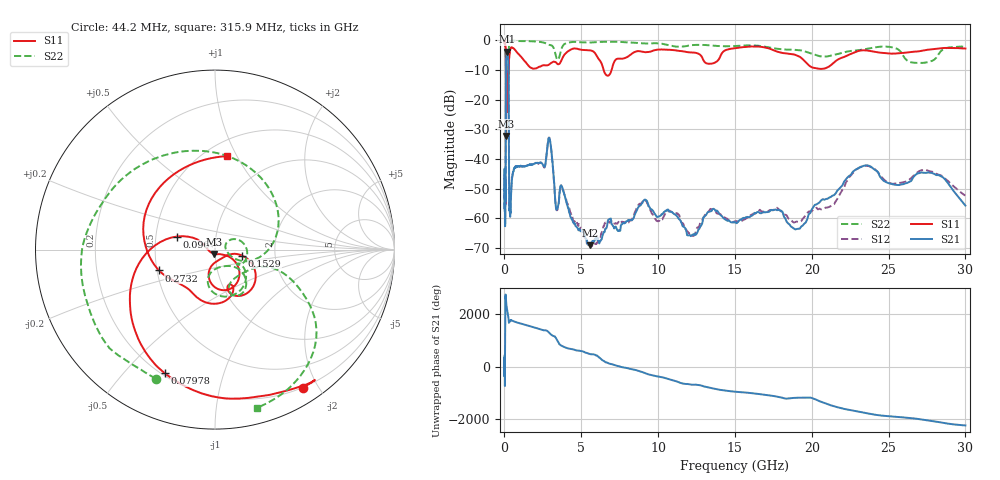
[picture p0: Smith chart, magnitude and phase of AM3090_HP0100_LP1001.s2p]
! Date/Time: Thu, Feb 28, 2019 1:57 PM
! Network Analyzer: Agilent Technologies E8364B Rev: A.07.50.67
! Sweep from 0.010 to 30.000 GHz, 1601 Points, Sweep Type: LOG
! Power Supply: 5.023 V, 0.002 A
# Hz S DB R 50
!freq MagS11 AngS11 MagS21 AngS21 MagS12 AngS12 MagS22 AngS22
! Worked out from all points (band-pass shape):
!   1601 points, 10 MHz to 30 GHz, reference 50 ohm
!   highest |S21| = -3.93 dB at 154.4 MHz (marker M1); lowest = -69.1 dB at 5.584 GHz (marker M2)
!   |S21| within 3 dB of the highest: 106 MHz to 249.3 MHz (143.4 MHz wide, 80.7 % of centre)
!   lowest |S11| = -32.2 dB at 104 MHz (marker M3), VSWR 1.05, Z = 49.5 - j2.38 ohm
!   |S11| at or under -10 dB: 94.42 MHz to 270.7 MHz (176.2 MHz wide, 96.5 % of centre); 6.454 GHz to 6.977 GHz (523.1 MHz wide, 7.79 % of centre)
!   |S22| runs from -24.6 to -0.1 dB; largest |S21 - S12| = 0.011
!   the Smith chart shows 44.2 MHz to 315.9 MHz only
!   S11 on the Smith chart (normalised r, x): 44.2 MHz: 0.19, -1.80; 79.78 MHz: 0.21, -0.65; 96 MHz: 0.64, +0.10; 152.9 MHz: 1.35, -0.09; 273.2 MHz: 0.51, -0.13; 315.9 MHz: 0.64, +0.91
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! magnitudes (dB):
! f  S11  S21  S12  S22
! 10 MHz  -0.3  -56.4  -46.5  -0.6
! 38.04 MHz  -0.5  -58.0  -61.1  -1.6
! 44.2 MHz  -0.8  -58.4  -59.2  -2.0
! 79.78 MHz  -2.6  -48.7  -50.1  -4.8
! 96 MHz  -13.0  -14.9  -14.8  -12.0
! 104 MHz  -32.2  -7.6  -7.6  -24.2
! 119.6 MHz  -12.7  -5.1  -5.0  -16.1
! 144.7 MHz  -23.7  -4.0  -4.0  -16.7
! 152.9 MHz  -16.2  -3.9  -3.9  -15.3
! 154.4 MHz  -15.1  -3.9  -3.9  -14.9
! 243.5 MHz  -10.9  -6.3  -6.3  -11.5
! 273.2 MHz  -9.6  -16.4  -16.3  -7.9
! 315.9 MHz  -5.6  -56.6  -55.5  -0.8
! 550.5 MHz  -2.7  -44.8  -44.7  -0.2
! 2.084 GHz  -9.5  -41.4  -41.4  -0.5
! 2.928 GHz  -8.2  -33.1  -33.0  -1.6
! 3.402 GHz  -7.8  -57.1  -57.3  -6.3
! 5.584 GHz  -3.5  -69.1  -68.8  -0.8
! 7.926 GHz  -5.9  -61.0  -61.0  -0.7
! 19.03 GHz  -5.2  -63.6  -61.1  -3.4
! 23.36 GHz  -3.4  -42.3  -42.4  -3.2
! 30 GHz  -2.8  -55.7  -52.3  -2.2
